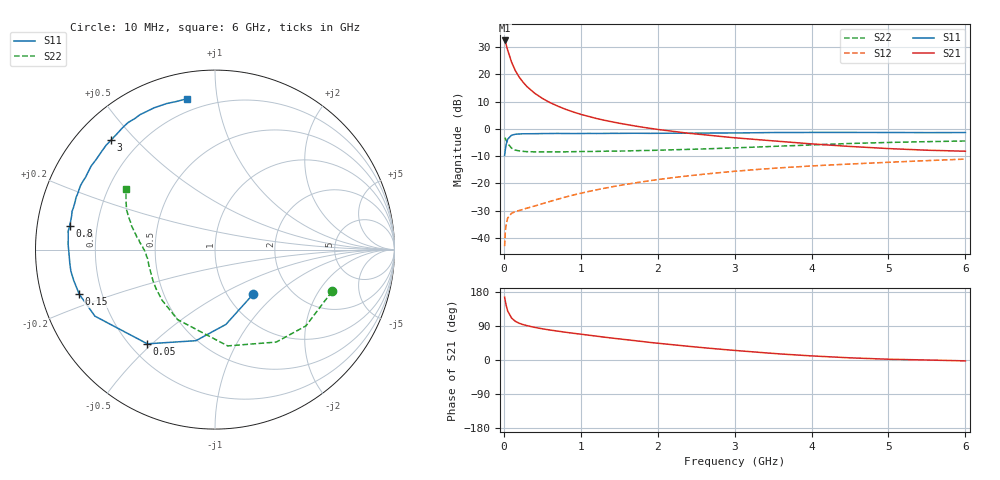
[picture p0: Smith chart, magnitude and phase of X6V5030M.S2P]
! SIEMENS Small Signal Semiconductors
! BFP193W
! Si NPN RF Bipolar Junction Transistor in SOT343
! VCE = 0.5 V  IC = 30 mA
! Common Emitter S-Parameters:  April 1994
# GHz  S  MA  R  50
!  f  S11  S21  S12  S22
! GHz  MAG  ANG  MAG  ANG  MAG  ANG  MAG  ANG
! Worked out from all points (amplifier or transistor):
!   40 points, 10 MHz to 6 GHz, reference 50 ohm
!   highest |S21| = 32.4 dB at 10 MHz (marker M1)
!   |S21| within 3 dB of that: start of sweep to 44.57 MHz
!   unconditionally stable (mu >= 1): 394.7 MHz to end of sweep
!   at 200 MHz: K = 0.62, MSG = 24.4 dB, |S12| = -29.9 dB
!   at 1.5 GHz: K = 1.43, MAG = 7.5 dB, |S12| = -20.8 dB
!   at 6 GHz: K = 1.22, MAG = -1.4 dB, |S12| = -11.1 dB
!   S11 on the Smith chart (normalised r, x): 10 MHz: 1.31, -0.73; 50 MHz: 0.27, -0.48; 150 MHz: 0.12, -0.16; 800 MHz: 0.10, +0.08; 3 GHz: 0.10, +0.43; 6 GHz: 0.13, +0.82
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0.01  0.3268 -49.3  41.53 165.8  0.0071 75.6  0.6921 -19.7
0.02  0.4212 -81.7  38.51 154.5  0.0134 64.1  0.6613 -40.0
0.03  0.5185 -101.8  34.99 144.3  0.0175 57.5  0.6179 -56.5
0.05  0.6463 -125.7  27.56 129.3  0.0233 44.5  0.5412 -82.5
0.1  0.7649 -151.0  16.72 110.9  0.0284 32.8  0.4422 -118.2
0.15  0.7959 -161.8  11.6 102.0  0.0306 30.5  0.4079 -136.3
0.2  0.8058 -167.7  8.834 97.0  0.032 31.4  0.394 -146.5
0.25  0.8119 -171.5  7.143 93.4  0.0335 32.8  0.3869 -152.9
0.3  0.8125 -174.4  5.95 90.7  0.0353 35.0  0.3821 -157.5
0.4  0.814 -178.6  4.494 86.1  0.0386 39.0  0.3788 -163.1
0.5  0.8188 177.9  3.616 82.4  0.0425 43.1  0.3786 -166.6
0.6  0.8202 175.5  3.021 79.1  0.0468 46.2  0.3783 -169.4
0.8  0.8207 170.7  2.287 73.3  0.0563 50.4  0.3792 -172.7
1  0.8205 166.8  1.841 68.1  0.0661 52.7  0.3839 -175.0
1.1  0.8243 165.1  1.692 65.5  0.0711 53.8  0.3848 -176.0
1.5  0.8261 157.9  1.267 55.7  0.0915 54.7  0.3918 -179.2
2.2  0.8323 146.1  0.9 40.2  0.1278 52.3  0.4135 175.9
3  0.8414 133.4  0.686 25.3  0.167 46.6  0.4484 169.3
3.2  0.8452 130.2  0.651 22.1  0.176 45.0  0.4589 167.8
4.5  0.8597 113.2  0.476 5.7  0.2269 34.5  0.5395 155.9
5.5  0.8528 104.7  0.406 0.0  0.2616 27.4  0.5822 148.4
6  0.8549 100.4  0.389 -2.3  0.2791 24.2  0.5991 145.4
